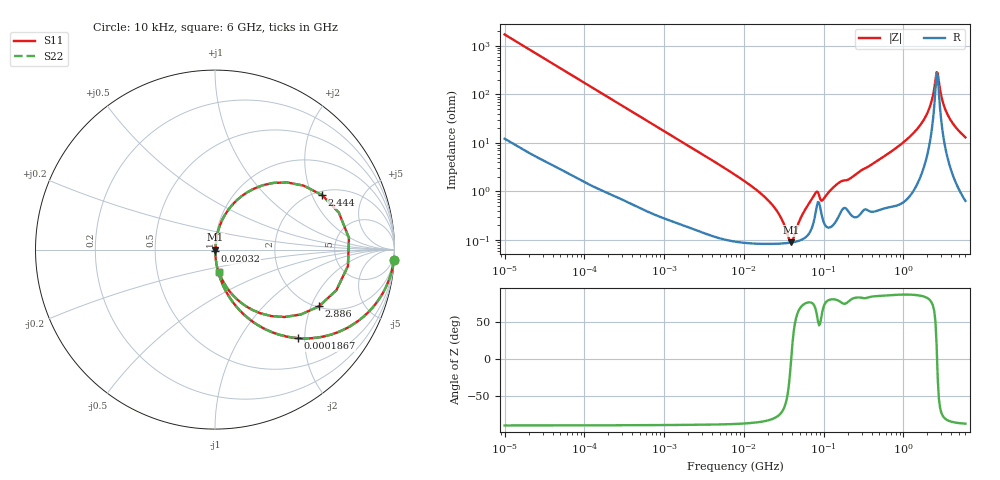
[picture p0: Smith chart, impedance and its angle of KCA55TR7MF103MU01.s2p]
!Murata Part Number: KCA55TR7MF103MU01
!These Parameters are Measured in Series Mode Connection
!Data Generated on Jan 08, 2026
!  o--ll--o
!Port1  Port2
!  o------o
!Operation Temp=25[degC], DC Bias Voltage=0[V]
!Freq. Start=10[kHz] Stop=6[GHz] 401[Steps]
# Hz S RI R 50
!Freq.(Hz) S11(Real) S11(Imag) S21(Real) S21(Imag) S12(Real) S12(Imag) S22(Real) S22(Imag)
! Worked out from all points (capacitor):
!   401 points, 10 kHz to 6 GHz, reference 50 ohm
!   read as one part in series: C = 9.32 nF near 10.69 kHz
!   lowest |Z| = 89.5 mohm at 39.53 MHz (marker M1)
!   series resonance near 39.24 MHz, so ESL is about 1.8 nH
!   S11 on the Smith chart (normalised r, x): 10 kHz: 1, -34; 186.7 kHz: 1.02, -1.85; 20.32 MHz: 1.00, -0.01; 2.444 GHz: 2.17, +2.38; 2.886 GHz: 2.04, -2.28; 6 GHz: 1.01, -0.26
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10000  0.9962 -0.0584  0.00385 0.0584  0.00385 0.0584  0.9962 -0.0584
40430  0.9458 -0.2225  0.0542 0.2225  0.0542 0.2225  0.9458 -0.2225
92862  0.7728 -0.4145  0.2272 0.4145  0.2272 0.4145  0.7728 -0.4145
186721  0.4621 -0.4934  0.5379 0.4934  0.5379 0.4934  0.4621 -0.4934
388143  0.17 -0.3695  0.83 0.3695  0.83 0.3695  0.17 -0.3695
862344  0.0421 -0.1934  0.9579 0.1934  0.9579 0.1934  0.0421 -0.1934
7745967  0.00141 -0.022  0.9986 0.022  0.9986 0.022  0.00141 -0.022
2.032318e7  0.000874 -0.00644  0.9991 0.00644  0.9991 0.00644  0.000874 -0.00644
2.741574e7  0.000854 -0.00336  0.9991 0.00336  0.9991 0.00336  0.000854 -0.00336
3.952748e7  0.000892 6.87e-05  0.9991 -6.87e-05  0.9991 -6.87e-05  0.000892 6.87e-05
7.193098e7  0.0019 0.00693  0.9981 -0.00693  0.9981 -0.00693  0.0019 0.00693
8.216701e7  0.00501 0.00853  0.995 -0.00853  0.995 -0.00853  0.00501 0.00853
9.70341e7  0.00281 0.00596  0.9972 -0.00596  0.9972 -0.00596  0.00281 0.00596
1.545823e8  0.00328 0.0147  0.9967 -0.0147  0.9967 -0.0147  0.00328 0.0147
6.67969e8  0.00854 0.0616  0.9915 -0.0616  0.9915 -0.0616  0.00854 0.0616
1.752557e9  0.0915 0.2437  0.9085 -0.2437  0.9085 -0.2437  0.0915 0.2437
2.139659e9  0.2631 0.3575  0.7369 -0.3575  0.7369 -0.3575  0.2631 0.3575
2.44414e9  0.5969 0.3037  0.4031 -0.3037  0.4031 -0.3037  0.5969 0.3037
2.612262e9  0.7462 0.0647  0.2538 -0.0647  0.2538 -0.0647  0.7462 0.0647
2.886376e9  0.5792 -0.3162  0.4208 0.3162  0.4208 0.3162  0.5792 -0.3162
3.643096e9  0.1447 -0.2957  0.8553 0.2957  0.8553 0.2957  0.1447 -0.2957
6e9  0.0227 -0.1264  0.9773 0.1264  0.9773 0.1264  0.0227 -0.1264
